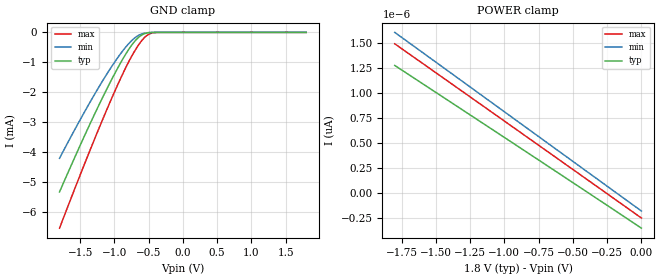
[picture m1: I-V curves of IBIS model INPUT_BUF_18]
| TEXAS INSTRUMENTS INCORPORATED
| Digital Light Processing Group
| IBIS Model of DLP4500FQE
| DLP4500FQE
| This file contains package information for the following:
|  LGA 80-pin S241 package as [Component] DLP4500_S241
| This device can be powered at the following Vccs:
|  2.5 volt Vcc
| This file provides unique models under the [Model Selector] for each Vcc.
| For operation at a specific Vcc, select the appropriate model after each
| [Model Selector] keyword.
[IBIS Ver]   3.2
[Comment char]  |_char
[File Name]   dlpm003.ibs
[File Rev]   2.0 | f_die
[Date]   January 09, 2014
[Source]   Data created from TI-SPICE simulations at TI-DLP.
[Notes]   The following is an IBIS list for the DLP4500FQE.
##notes##|
[Disclaimer] Property of Texas Instruments Incorporated.  Unauthorized
   reproduction and/or distribution is strictly prohibited.
   This product is protected under copyright law.
   Created  2013, (C) Copyright  2013, Texas Instruments
   Incorporated, All Rights Reserved
   UNLESS THERE IS A SIGNED, WRITTEN AGREEMENT TO THE
   CONTRARY, TEXAS INSTRUMENTS (TI) IS PROVIDING THE IBIS
   MODELS  AND WITHOUT ANY WARRANTY, EXPRESSED OR
   IMPLIED.  TI assumes no liability for:
   1) the accuracy of the IBIS models provided to your
   company;
   2) the proper functioning of these IBIS Models in your
   design or for any resulting applications; or
   3) infringement of patents, copyrights or intellectual
   property rights resulting from your use of these IBIS
   models.
   TI provides IBIS Models as a service to our customers.
   You and your company shall not distribute, sell or give
   these models to anyone else without prior written
   permission from TI.
   TI reserves the right to make changes to our products or
   to discontinue any semiconductor product or service
   without notice, and advises our customers to obtain the
   latest version of relevant information to verify, before
   placing orders, that the information being relied on is
   current.
   Please be aware that your receipt and use of the IBIS
   information provided shall serve as acceptance of these
   terms and conditions.  If you do not accept these terms,
   you should return or destroy the IBIS models and any
   other accompanying information immediately.
| Component DLP4500_S241 80-pin LGA
[Component]   DLP4500_S241
[Manufacturer]   Texas Instruments, Inc.
[Package]
|   typ   min   max
R_pkg   1.107E+00   5.976E-01   1.318E+00
L_pkg   9.495E-09   5.447E-09   1.351E-08
C_pkg   2.933E-12   1.650E-12   3.894E-12
[Pin]   signal_name   model_name   R_pin   L_pin   C_pin
C1   VCC   POWER
C2   VCC   POWER
C3   DATA(6)   INPUT_BUF   1.076E+00   5.984E-09   2.630E-12
C4   DATA(4)   INPUT_BUF   1.129E+00   6.655E-09   2.861E-12
C5   VSS   GND
C6   DATA(5)   INPUT_BUF   1.054E+00   6.292E-09   2.834E-12
C7   DATA(3)   INPUT_BUF   1.063E+00   7.762E-09   2.836E-12
C8   VSS   GND
C9   DATA(2)   INPUT_BUF   1.086E+00   8.753E-09   2.801E-12
C10   DATA(1)   INPUT_BUF   1.088E+00   9.656E-09   2.941E-12
C11   VSS   GND
C12   DATA(0)   INPUT_BUF   1.130E+00   1.041E-08   2.754E-12
C13   DATA(7)   INPUT_BUF   1.091E+00   9.445E-09   3.046E-12
C14   VSS   GND
C15   DATA(8)   INPUT_BUF   1.121E+00   1.009E-08   2.961E-12
C16   DATA(9)   INPUT_BUF   1.103E+00   1.025E-08   2.998E-12
C17   VSS   GND
C18   DATA(10)   INPUT_BUF   1.129E+00   1.151E-08   3.014E-12
C19   DATA(11)   INPUT_BUF   1.122E+00   1.143E-08   3.493E-12
C20   VSS   GND
C21   DATA(12)   INPUT_BUF   1.291E+00   1.330E-08   3.294E-12
C22   DATA(13)   INPUT_BUF   1.318E+00   1.339E-08   3.675E-12
C23   VSS   GND
C24   VSS   GND
C25   VREF   POWER
C26   VREF   POWER
C27   VSS   GND
C28   VSS   GND
C29   DRC_BUS   INPUT_BUF   1.138E+00   1.022E-08   3.185E-12
C30   VSS   GND
C31   VBIAS   POWER
C32   VBIAS   POWER
C33   DRC_OEZ   INPUT_BUF   5.976E-01   5.545E-09   1.825E-12
C34   VCC   POWER
C35   VCC   POWER
C36   DRC_STROBE INPUT_BUF   1.252E+00   7.652E-09   2.664E-12
C37   VCC   POWER
C38   VCC   POWER
C39   VCC   POWER
C40   VCC   POWER
D1   VCC   POWER
D2   VCC   POWER
D3   TRC   INPUT_BUF   7.360E-01   5.447E-09   1.650E-12
D4   DATA(17)   INPUT_BUF   1.081E+00   6.800E-09   3.207E-12
D5   VSS   GND
D6   DATA(20)   INPUT_BUF   1.159E+00   6.901E-09   2.413E-12
D7   DATA(22)   INPUT_BUF   1.078E+00   7.570E-09   2.368E-12
D8   VSS   GND
D9   DATA(18)   INPUT_BUF   1.091E+00   8.243E-09   2.958E-12
D10   DATA(19)   INPUT_BUF   1.095E+00   9.298E-09   3.231E-12
D11   VSS   GND
D12   LOADB   INPUT_BUF   1.195E+00   1.042E-08   2.999E-12
D13   DCLK   INPUT_BUF   1.182E+00   1.064E-08   3.009E-12
D14   VSS   GND
D15   DATA(23)   INPUT_BUF   1.202E+00   1.080E-08   3.206E-12
D16   DATA(21)   INPUT_BUF   1.267E+00   1.222E-08   3.378E-12
D17   VSS   GND
D18   SCTRL   INPUT_BUF   1.304E+00   1.304E-08   3.569E-12
D19   DATA(16)   INPUT_BUF   1.121E+00   1.153E-08   3.274E-12
D20   VSS   GND
D21   DATA(15)   INPUT_BUF   1.210E+00   1.275E-08   3.169E-12
D22   DATA(14)   INPUT_BUF   1.310E+00   1.351E-08   3.894E-12
D23   VSS   GND
D24   VSS   GND
D25   VOFFSET   POWER
D26   VOFFSET   POWER
D27   VSS   GND
D28   VSS   GND
D29   SAC_CLK   INPUT_BUF   1.124E+00   1.140E-08   3.108E-12
D30   VSS   GND
D31   VRESET   POWER
D32   VRESET   POWER
D33   SAC_BUS   INPUT_BUF   9.075E-01   8.239E-09   2.610E-12
D34   VCC   POWER
D35   VCC   POWER
D36   NO_CONNECT NC
D37   VCC   POWER
D38   VCC   POWER
D39   VCC   POWER
D40   VCC   POWER
| Model INPUT_BUF
[Model Selector]   INPUT_BUF
INPUT_BUF_18   1.8 volt Vcc
| Models and submodels in the file (1): INPUT_BUF_18 (Input)
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[Model]   INPUT_BUF_18
Model_type  Input
Vinl=0.36
Vinh=1.44
| variable   typ   min   max
C_comp   0.29pF   0.23pF   0.31pF
[Temperature Range]   40   100   0
| Ambient temperature   25   85   -40
[Voltage range]   1.8   1.65   1.95
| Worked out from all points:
|   GND clamp passes 1 mA (typ) near -0.90 V on its own axis
[GND Clamp]
| INPUT_BUF_18
|   Voltage   I(typ)   I(min)   I(max)
-1.8V     -5.319mA   -4.198mA   -6.527mA
-1.545V   -4.001mA   -3.106mA   -5.023mA
-1.32V    -2.88mA    -2.189mA   -3.733mA
-1.12V    -1.934mA   -1.427mA   -2.63mA
-950mV    -1.186mA   -840.2uA   -1.741mA
-820mV    -673.5uA   -453.5uA   -1.113mA
-715mV    -332.5uA   -209.4uA   -667.5uA
-625mV    -127.6uA   -75.21uA   -349uA
-535mV    -27.06uA   -17.14uA   -121.4uA
-460mV    -4.641uA   -3.582uA   -29.58uA
-355mV    -235.9nA   -285.7nA   -1.811uA
1.8V      14.91pA    62.54pA    31.07pA
[POWER Clamp]
| INPUT_BUF_18
|   Voltage   I(typ)   I(min)   I(max)
-1.8V     1.275pA    1.605pA    1.491pA
-830mV    403.9fA    644.9fA    556.4fA
-405mV    19.82fA    224fA      145.4fA
-16.28fV  -347.9fA   -177.3fA   -247.1fA
